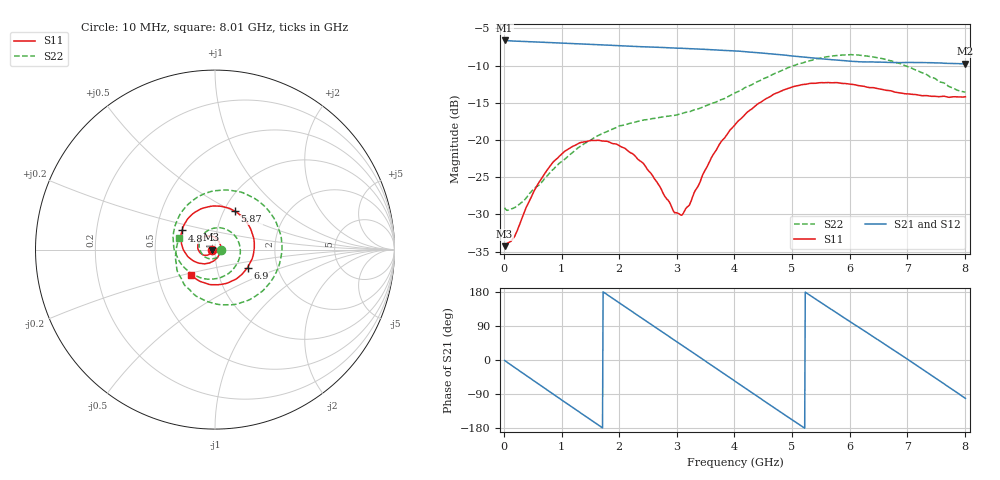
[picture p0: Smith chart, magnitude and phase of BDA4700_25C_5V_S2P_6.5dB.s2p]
!Agilent Technologies,E5071B,MY42404982,A.09.10
!Date: Mon Oct 20 13:29:12 2025
!Data & Calibration Information:
!Freq	S11:SOLT2(ON)	S21:SOLT2(ON)	S12:SOLT2(ON)	S22:SOLT2(ON)
# Hz S RI R 50
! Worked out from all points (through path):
!   801 points, 10 MHz to 8.01 GHz, reference 50 ohm
!   highest |S21| = -6.61 dB at 10 MHz (marker M1); lowest = -9.8 dB at 8.01 GHz (marker M2)
!   group delay of S21, straight-line fit = 284 ps
!   lowest |S11| = -34.3 dB at 10 MHz (marker M3), VSWR 1.04, Z = 48.1 - j0.0911 ohm
!   |S11| at or under -10 dB: start of sweep to end of sweep
!   |S22| runs from -29.5 to -8.5 dB; largest |S21 - S12| = 0.0037
!   S11 on the Smith chart (normalised r, x): 10 MHz: 0.96, -0.00; 4.8 GHz: 0.68, +0.15; 5.87 GHz: 1.13, +0.51; 6.9 GHz: 1.41, -0.29; 8.01 GHz: 0.74, -0.22
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1e7  -0.0193 -0.000946  0.467 -0.00999  0.467 -0.0106  0.035 -0.0028
3.3e8  -0.0247 -0.019  0.3757 -0.2655  0.3756 -0.2657  0.0228 -0.0312
7.1e8  -0.0503 -0.0322  0.1165 -0.4383  0.1163 -0.4386  -0.0194 -0.0518
1.02e9  -0.0789 -0.0217  -0.1345 -0.4276  -0.135 -0.4276  -0.0644 -0.0335
1.35e9  -0.096 0.00982  -0.3478 -0.2733  -0.348 -0.2734  -0.0884 0.0256
1.64e9  -0.0895 0.044  -0.4329 -0.0616  -0.4329 -0.0616  -0.0651 0.0855
1.93e9  -0.0637 0.0694  -0.4008 0.1611  -0.401 0.1615  -0.000987 0.1203
2.32e9  -0.0158 0.0728  -0.1992 0.3757  -0.1993 0.3758  0.0986 0.0898
2.68e9  0.0212 0.0457  0.0657 0.4149  0.0659 0.4147  0.1412 -0.00751
2.95e9  0.0314 0.00983  0.2487 0.3331  0.2485 0.3326  0.117 -0.0874
3.1e9  0.0293 -0.012  0.3268 0.2531  0.3261 0.254  0.0858 -0.1246
3.54e9  -0.0137 -0.0665  0.4029 -0.0522  0.4026 -0.0529  -0.0543 -0.1632
4.01e9  -0.1056 -0.07  0.2229 -0.3285  0.223 -0.3283  -0.1943 -0.0713
4.39e9  -0.1731 -0.00774  -0.0341 -0.3851  -0.0343 -0.386  -0.2336 0.077
4.8e9  -0.1834 0.1068  -0.2752 -0.2541  -0.274 -0.2551  -0.1567 0.2452
5.35e9  -0.0659 0.2313  -0.3472 0.0813  -0.3477 0.0804  0.1086 0.3267
5.87e9  0.1108 0.213  -0.1437 0.3112  -0.1433 0.3109  0.3385 0.1558
6.25e9  0.1989 0.115  0.0722 0.3268  0.0757 0.3259  0.3631 -0.0651
6.68e9  0.2124 -0.033  0.274 0.1883  0.2748 0.1879  0.2228 -0.2613
6.9e9  0.1812 -0.0999  0.3235 0.0725  0.3238 0.0708  0.1079 -0.3058
7.48e9  0.022 -0.1954  0.2264 -0.2403  0.2264 -0.2411  -0.1713 -0.195
8.01e9  -0.1326 -0.1434  -0.0642 -0.3189  -0.0642 -0.3194  -0.1996 0.0655
